(* Logix 5000 AddOnInstructionDefinition export EH_Micropilot_FMR43_IOL; software revision 38.00 *)

TYPE EH_CommAOI_Data :
STRUCT
   Device_Comm_Error : BOOL;
   CommSuccess : BOOL;
   CommFailed : BOOL;
   CommTimeOut : BOOL;
   StateDone : BOOL;
   NewState : BOOL;
   OldState : SINT;
   PortSize : SINT;
   DevicePort : SINT;
   MaxState : SINT;
   State : SINT;
   VendorID : INT;
   DeviceID : DINT;
   CyclicData : INT[16];
   AcyclicData : DINT[8];
   ReplayIndex : INT;
   AOI_Diagnostic : DINT;
   ConnectionStatus : DINT;
   OutputData : INT[16];
END_STRUCT
END_TYPE

ADD_ON_INSTRUCTION EH_Micropilot_FMR43_IOL   (* revision 1.2, vendor Endress+Hauser *)
// Micropilot FMR 43  Rev 1 IO-Link
// Revision note:
// 1.2 Added HeartbeatVerification, fixed Foamfunction
// 1.1 Changed the Datatype from Unsigned to Signed
// Add Disconnect check
VAR_IN_OUT
   DataToSend : INT[10]; {required}
   CommAOIBusy : DINT; {required}
   ActiveComPort : DINT; {required}
   DeviceAOISendRequest : DINT; {required}
   CommError : INT; {required}
   DeviceData : EH_CommAOI_Data; {required}
END_VAR
VAR_INPUT
   iSetSimulation : BOOL; {visible}
   iSimulationVariable : INT; {visible}
   iSimulationValue_Level : REAL; {visible}
   iSimulationValue_Distance : REAL; {visible}
   iSetUnit : BOOL; {visible}
   iUnit : SINT; {visible}
   iFoamDetection_Update : BOOL; {visible}
   iStart_HeartbeatVerification : BOOL; {visible}
END_VAR
VAR_OUTPUT
   qVendor_ID : DINT; {access Read Only, visible}
   qDevice_ID : DINT; {access Read Only, visible}
   qLevelLinearized : REAL; {access None, visible}
   qDistance : REAL; {visible}
   qExtendedDeviceStatus : INT; {access Read Only, visible}
   qUnit : SINT; {access Read Only, visible}
   qFoamIndex : REAL; {access Read Only, visible}
   qFoamDetected : BOOL; {access Read Only, visible}
   qBuildupIndex : REAL; {access Read Only, visible}
   qBuildupDetected : BOOL; {access Read Only, visible}
   qSSC1_1 : BOOL; {access Read Only, visible}
   qSSC1_2 : BOOL; {access Read Only, visible}
   qSSC2_1 : BOOL; {access Read Only, visible}
   qSSC2_2 : BOOL; {access Read Only, visible}
   qVerificationID : INT; {visible}
   qPassed : BOOL; {visible}
   qFailed : BOOL; {visible}
   qAOI_Diagnostic : DINT; {access Read Only, visible}
END_VAR
VAR_IN_OUT
   qAOI_Diagnostic_String : STRING; {required}
END_VAR
VAR_OUTPUT
   qActual_Diagnostics_Code : DINT; {access Read Only, visible}
END_VAR
VAR_IN_OUT
   qActual_Diagnostics_String : STRING; {required}
END_VAR
VAR_OUTPUT
   qLast_Diagnostics_Code : DINT; {visible}
END_VAR
VAR_IN_OUT
   qLast_Diagnostics_String : STRING; {required}
END_VAR
VAR_OUTPUT
   qCommError : DINT; {access None}
   qCommunicationBusy : DINT; {access Read Only, visible}
   qDeviceConnectionError : BOOL; {access Read Only, visible}
END_VAR
VAR
   Temp_DINT : DINT; {access None}
   CMD_Index : INT; {access None}
   CMD_Subindex : INT; {access None}
   CMD_ByteLength : INT; {access None}
   oldCondStatus : INT; {access None}
   oldSetSimulation : SINT; {access None}
   SetSimulation : SINT; {access None}
   SetUnit : SINT; {access None}
   oldSetUnit : SINT; {access None}
   Trigger : BOOL; {access None}
   CMD_Rd : BOOL; {access None}
   CMD_Wr : BOOL; {access None}
   SimulationDINT : DINT; {access None}
   InputByteLength : DINT; {access None}
   AOI_Prio : BOOL; {access None}
   StateMin : DINT; {access None}
   firstTimeDone : BOOL; {access None}
   OldStatus : DINT; {access None}
   CondStatusChanged : BOOL; {access None}
   Calc_ExtendedDeviceStatus : DINT; {access None}
   Totalizer1_DINT : DINT; {access None}
   SimActive : BOOL; {access None}
   CondStatusActive : BOOL; {access None}
   ActiveAOI : BOOL; {access None}
   Skip : BOOL; {access None}
   SimChanged : BOOL; {access None}
   UnitActive : BOOL; {access None}
   UnitChanged : BOOL; {access None}
   DeviceID : DINT; {access None}
   Calc_LevelLin : DINT; {access None}
   Calc_Distance : DINT; {access None}
   FALSE : BOOL; {access None}
   TRUE : BOOL := 1; {access None}
   temp_string1 : STRING; {access None}
   temp_string2 : STRING; {access None}
   qFoamIndexDINT : DINT; {access None}
   qFoamDetectedDINT : DINT; {access None}
   qBuildupIndexDINT : DINT; {access None}
   qBuildupDetectedDINT : DINT; {access None}
   qFoamDetectedREAL : REAL; {access None}
   qBuildupDetectedREAL : REAL; {access None}
   qLevelLinearizedTemp : REAL; {access None}
   TempLevel_DINT : DINT; {access None}
   TempDistance_DINT : DINT; {access None}
   qDistanceTemp : REAL; {access None}
   init : BOOL; {access None}
   SkipStep2 : BOOL; {access None}
   rTempLevel : REAL; {access None}
   rTempDistance : REAL;
   Start_HeartbeatVerification : SINT; {access None}
   oldStart_HeartbeatVerification : SINT; {access None}
   HeartbeatVerificationChanged : BOOL; {access None}
   HeartbeatVerificationActive : BOOL; {access None}
END_VAR

ROUTINE Logic   (* structured text *)
// Picomag Communication via AL1323
   // =======================================================================
   // Endress+Hauser Digital Solutions
   // ©Copyright (2024) All Rights Reserved
   // =======================================================================
   // Name:                EH_Micropilot_FMR43_IOL
   // Version:             1.2
   // Datum:               11.2025
   // Library:             01.01.00
   // Engineering:         Studio5000 V38.00.00
   // Author:              EH
   // =======================================================================
   
   qAOI_Diagnostic := DeviceData.AOI_Diagnostic;
   qCommunicationBusy := CommAOIBusy;
   DeviceID := 9553409;
   StateMin := 0;
   DeviceData.MaxState := 98;
   
   if DeviceData.DevicePort = 0 or DeviceData.DeviceID <> DeviceID or DeviceData.ConnectionStatus <> 1 then
   
   	qVendor_ID := DeviceData.VendorID;
   	qDevice_ID := DeviceData.DeviceID;
   	qLevelLinearized	:= 0;
   	qDistance	:= 0;
   	qExtendedDeviceStatus	:= 0;
   	qUnit	:= 0;
   	qFoamIndex := 0;   // Foam index
   	qFoamDetected := FALSE;   // Foam detection - TRUE if foam detected
   	qBuildupIndex := 0;   // Buildup index
   	qBuildupDetected := FALSE;   // Buildup detection - TRUE if buildup detected
   	qSSC1_1	:= FALSE;
   	qSSC1_2	:= FALSE;
   	qSSC2_1	:= FALSE;
   	qSSC2_2	:= FALSE;
   	qPassed := FALSE;
   	qFailed := FALSE;
   	qVerificationID := 0;
   	qPassed := FALSE;
   	qFailed	:= FALSE;
   	qActual_Diagnostics_Code	:= 0;
   	qLast_Diagnostics_Code	:= 0;
   	qLast_Diagnostics_String	:= '';
   	oldCondStatus := 0;
   	CondStatusChanged := FALSE;
   	init := FALSE;
   
   	if DeviceData.DevicePort = 0 then
   
   		qActual_Diagnostics_String	:= 'Device Port is Zero';
   		DeviceData.AOI_Diagnostic.1 := TRUE;
   
   	elsif DeviceData.ConnectionStatus <> 1 then
   
   		qActual_Diagnostics_String	:= 'No Device connected';
   		qDeviceConnectionError := TRUE;
   
   	elsif DeviceData.DeviceID <> DeviceID then
   
   		qActual_Diagnostics_String	:= 'Wrong DeviceID';
   		DeviceData.AOI_Diagnostic.2 := TRUE;
   	end_if;
   
   else
   
   	if qActual_Diagnostics_Code = 0  then
   
   		qActual_Diagnostics_String	:= '--------';
   
   	end_if;
   
   	if qLast_Diagnostics_Code = 0 then
   
   		qLast_Diagnostics_String	:= '--------';
   
   	end_if;
   
   	DeviceData.AOI_Diagnostic.1 := FALSE;
   	qDeviceConnectionError := FALSE;
   	DeviceData.AOI_Diagnostic.2  := FALSE;
   
   end_if;
   
   // Case device disconnected during communication to avoid blocking the communication
   if (DeviceData.AOI_Diagnostic.0 or qDeviceConnectionError or DeviceData.AOI_Diagnostic.2) and ActiveAOI and ActiveComPort = DeviceData.DevicePort and CommAOIBusy = 1 then
   
   	DeviceData.State := 0;
   	CommAOIBusy := 0;
   	DeviceAOISendRequest.[DeviceData.DevicePort] := 0;
   	ActiveComPort := 0;
   	ActiveAOI := 0;
   	DataToSend[0] := 0;
   	DataToSend[1] := 0;
   	DataToSend[2] := 0;
   	DataToSend[3] := 0;
   	DataToSend[4] := 0;
   	DataToSend[5] := 0;
   	DataToSend[6] := 0;
   	DataToSend[7] := 0;
   	DataToSend[8] := 0;
   	DataToSend[9] := 0;
   	DeviceData.StateDone := FALSE;
   	DeviceData.NewState := FALSE;
   	DeviceData.OldState := 0;
   	ActiveAOI := FALSE;
   
   end_if;
   
   if not DeviceData.AOI_Diagnostic.0
   	and not qDeviceConnectionError
   	and not DeviceData.AOI_Diagnostic.2
   	and DeviceData.DevicePort > 0 then
   
   	//*********************************
   	//Vendor ID
   	//*********************************
   
   		qVendor_ID := DeviceData.VendorID;
   
   	//*********************************
   	//Device ID
   	//*********************************
   
   		qDevice_ID := DeviceData.DeviceID;
   
   	//*********************************
   	// FMR43
   	//*********************************
   
   		Calc_LevelLin				:= 0;
   		Calc_Distance				:= 2;
   		Calc_ExtendedDeviceStatus	:= 4;
   
   	//*********************************
   	//Process Data Level Linearized
   	//*********************************
   
   		TempLevel_DINT	 := DeviceData.CyclicData[Calc_LevelLin+1];
   		TempLevel_DINT.8	 := DeviceData.CyclicData[Calc_LevelLin+1].8;
   		TempLevel_DINT.9  := DeviceData.CyclicData[Calc_LevelLin+1].9;
   		TempLevel_DINT.10 := DeviceData.CyclicData[Calc_LevelLin+1].10;
   		TempLevel_DINT.11 := DeviceData.CyclicData[Calc_LevelLin+1].11;
   		TempLevel_DINT.12 := DeviceData.CyclicData[Calc_LevelLin+1].12;
   		TempLevel_DINT.13 := DeviceData.CyclicData[Calc_LevelLin+1].13;
   		TempLevel_DINT.14 := DeviceData.CyclicData[Calc_LevelLin+1].14;
   		TempLevel_DINT.15 := DeviceData.CyclicData[Calc_LevelLin+1].15;
   		TempLevel_DINT.16 := DeviceData.CyclicData[Calc_LevelLin].0;
   		TempLevel_DINT.17 := DeviceData.CyclicData[Calc_LevelLin].1;
   		TempLevel_DINT.18 := DeviceData.CyclicData[Calc_LevelLin].2;
   		TempLevel_DINT.19 := DeviceData.CyclicData[Calc_LevelLin].3;
   		TempLevel_DINT.20 := DeviceData.CyclicData[Calc_LevelLin].4;
   		TempLevel_DINT.21 := DeviceData.CyclicData[Calc_LevelLin].5;
   		TempLevel_DINT.22 := DeviceData.CyclicData[Calc_LevelLin].6;
   		TempLevel_DINT.23 := DeviceData.CyclicData[Calc_LevelLin].7;
   		TempLevel_DINT.24 := DeviceData.CyclicData[Calc_LevelLin].8;
   		TempLevel_DINT.25 := DeviceData.CyclicData[Calc_LevelLin].9;
   		TempLevel_DINT.26 := DeviceData.CyclicData[Calc_LevelLin].10;
   		TempLevel_DINT.27 := DeviceData.CyclicData[Calc_LevelLin].11;
   		TempLevel_DINT.28 := DeviceData.CyclicData[Calc_LevelLin].12;
   		TempLevel_DINT.29 := DeviceData.CyclicData[Calc_LevelLin].13;
   		TempLevel_DINT.30 := DeviceData.CyclicData[Calc_LevelLin].14;
   		TempLevel_DINT.31 := DeviceData.CyclicData[Calc_LevelLin].15;
   
   		COP(TempLevel_DINT,qLevelLinearizedTemp,1);
   
   	//*********************************
   	//Process Data Distance
   	//*********************************
   
   		TempDistance_DINT	 := DeviceData.CyclicData[Calc_Distance+1];
   		TempDistance_DINT.8	 := DeviceData.CyclicData[Calc_Distance+1].8;
   		TempDistance_DINT.9	 := DeviceData.CyclicData[Calc_Distance+1].9;
   		TempDistance_DINT.10 := DeviceData.CyclicData[Calc_Distance+1].10;
   		TempDistance_DINT.11 := DeviceData.CyclicData[Calc_Distance+1].11;
   		TempDistance_DINT.12 := DeviceData.CyclicData[Calc_Distance+1].12;
   		TempDistance_DINT.13 := DeviceData.CyclicData[Calc_Distance+1].13;
   		TempDistance_DINT.14 := DeviceData.CyclicData[Calc_Distance+1].14;
   		TempDistance_DINT.15 := DeviceData.CyclicData[Calc_Distance+1].15;
   		TempDistance_DINT.16 := DeviceData.CyclicData[Calc_Distance].0;
   		TempDistance_DINT.17 := DeviceData.CyclicData[Calc_Distance].1;
   		TempDistance_DINT.18 := DeviceData.CyclicData[Calc_Distance].2;
   		TempDistance_DINT.19 := DeviceData.CyclicData[Calc_Distance].3;
   		TempDistance_DINT.20 := DeviceData.CyclicData[Calc_Distance].4;
   		TempDistance_DINT.21 := DeviceData.CyclicData[Calc_Distance].5;
   		TempDistance_DINT.22 := DeviceData.CyclicData[Calc_Distance].6;
   		TempDistance_DINT.23 := DeviceData.CyclicData[Calc_Distance].7;
   		TempDistance_DINT.24 := DeviceData.CyclicData[Calc_Distance].8;
   		TempDistance_DINT.25 := DeviceData.CyclicData[Calc_Distance].9;
   		TempDistance_DINT.26 := DeviceData.CyclicData[Calc_Distance].10;
   		TempDistance_DINT.27 := DeviceData.CyclicData[Calc_Distance].11;
   		TempDistance_DINT.28 := DeviceData.CyclicData[Calc_Distance].12;
   		TempDistance_DINT.29 := DeviceData.CyclicData[Calc_Distance].13;
   		TempDistance_DINT.30 := DeviceData.CyclicData[Calc_Distance].14;
   		TempDistance_DINT.31 := DeviceData.CyclicData[Calc_Distance].15;
   
   		COP(TempDistance_DINT,qDistanceTemp,1);
   
   		case qUnit of
   
   				//*********************************
   				45: // m
   				//*********************************
   					qDistance := qDistanceTemp;
   					qLevelLinearized := qLevelLinearizedTemp;
   
   				//*********************************
   				47: // inch
   				//*********************************
   					qDistance := qDistanceTemp * 39.37007874;
   					qLevelLinearized := qLevelLinearizedTemp * 39.37007874;
   
   				//*********************************
   				49: // mm
   				//*********************************
   					qDistance := qDistanceTemp * 1000;
   					qLevelLinearized := qLevelLinearizedTemp * 1000;
   
   				else // Base unit
   					qDistance := qDistanceTemp;
   					qLevelLinearized := qLevelLinearizedTemp;
   
   			end_case;
   
   	//*********************************
   	// Extended device Status
   	//*********************************
   
   		qExtendedDeviceStatus.0 := DeviceData.CyclicData[Calc_ExtendedDeviceStatus].8;
   		qExtendedDeviceStatus.1 := DeviceData.CyclicData[Calc_ExtendedDeviceStatus].9;
   		qExtendedDeviceStatus.2 := DeviceData.CyclicData[Calc_ExtendedDeviceStatus].10;
   		qExtendedDeviceStatus.3 := DeviceData.CyclicData[Calc_ExtendedDeviceStatus].11;
   		qExtendedDeviceStatus.4 := DeviceData.CyclicData[Calc_ExtendedDeviceStatus].12;
   		qExtendedDeviceStatus.5 := DeviceData.CyclicData[Calc_ExtendedDeviceStatus].13;
   		qExtendedDeviceStatus.6 := DeviceData.CyclicData[Calc_ExtendedDeviceStatus].14;
   		qExtendedDeviceStatus.7 := DeviceData.CyclicData[Calc_ExtendedDeviceStatus].15;
   
   	//*********************************
   	// Process Parameter SSC
   	//*********************************
   
   		qSSC1_1 := DeviceData.CyclicData[Calc_ExtendedDeviceStatus].0;
   		qSSC1_2 := DeviceData.CyclicData[Calc_ExtendedDeviceStatus].1;
   
   		qSSC2_1 := DeviceData.CyclicData[Calc_ExtendedDeviceStatus].2;
   		qSSC2_2 := DeviceData.CyclicData[Calc_ExtendedDeviceStatus].3;
   
   	//*********************************
   	// Checking for Changed Status
   	//*********************************
   
   		SetSimulation.0 := iSetSimulation;
   		SetUnit.0 := iSetUnit;
   		Start_HeartbeatVerification.0 := iStart_HeartbeatVerification;
   
   	if oldCondStatus <> qExtendedDeviceStatus and not CondStatusChanged or iFoamDetection_Update and (qExtendedDeviceStatus = 120 or qExtendedDeviceStatus = 121) then
   
   		CondStatusChanged := TRUE;
   		oldCondStatus := qExtendedDeviceStatus;
   
   	end_if;
   
   	if oldSetSimulation <> SetSimulation and not SimChanged then
   
   		if oldSetSimulation < SetSimulation then
   
   			SimChanged := TRUE;
   
   		end_if;
   
   		oldSetSimulation := SetSimulation;
   
   	end_if;
   
   	if oldSetUnit <> SetUnit and not UnitChanged then
   
   		if oldSetUnit < SetUnit then
   
   			UnitChanged := TRUE;
   
   		end_if;
   
   		oldSetUnit := SetUnit;
   
   	end_if;
   
   	if oldStart_HeartbeatVerification <> Start_HeartbeatVerification and not HeartbeatVerificationChanged then
   
   		if oldStart_HeartbeatVerification < Start_HeartbeatVerification then
   
   			HeartbeatVerificationChanged := TRUE;
   
   		end_if;
   
   		oldStart_HeartbeatVerification := Start_HeartbeatVerification;
   
   	end_if;
   
   	if CondStatusChanged
   	and not ActiveAOI
   	and not CondStatusActive
   	and not Skip then
   
   		DeviceAOISendRequest.[DeviceData.DevicePort] := TRUE;
   		CondStatusActive := TRUE;
   		Skip := TRUE;
   
   	elsif SimChanged
   		and not ActiveAOI
   		and not SimActive
   		and not Skip then
   
   		DeviceAOISendRequest.[DeviceData.DevicePort] := TRUE;
   		SimActive := TRUE;
   		Skip := TRUE;
   
   	elsif HeartbeatVerificationChanged
   		and not ActiveAOI
   		and not HeartbeatVerificationActive
   		and not Skip then
   
   		DeviceAOISendRequest.[DeviceData.DevicePort] := TRUE;
   		HeartbeatVerificationActive := TRUE;
   		Skip := TRUE;
   
   	elsif UnitChanged
   		and not ActiveAOI
   		and not UnitActive
   		and not Skip then
   
   		DeviceAOISendRequest.[DeviceData.DevicePort] := TRUE;
   		UnitActive := TRUE;
   		Skip := TRUE;
   
   	end_if;
   
   	if ActiveComPort = DeviceData.DevicePort then
   
   		AOI_Prio := TRUE;
   
   	else
   
   		AOI_Prio := FALSE;
   
   	end_if;
   
   	if (SimActive or UnitActive or HeartbeatVerificationActive or CondStatusActive) and CommAOIBusy = 1  and DeviceData.State = 0 and AOI_Prio and not ActiveAOI then
   
   		ActiveAOI := TRUE;
   		Skip := FALSE;
   
   	end_if;
   
   	qCommunicationBusy := CommAOIBusy;
   	qAOI_Diagnostic :=DeviceData.AOI_Diagnostic;
   
   	//*********************************
   	// States for Execution
   	//*********************************
   
   	if ActiveAOI or DeviceData.State = DeviceData.MaxState then
   
   	case DeviceData.State of
   
   		//*********************************
   		0: // Idle
   		//*********************************
   
   			// Initializing
   			Trigger := 0;
   			CMD_Index := 0;
   			CMD_Subindex := 0;
   			CMD_Wr := FALSE;
   			CMD_Rd := FALSE;
   		    CMD_ByteLength := 0;
   
   			if DeviceData.DevicePort = ActiveComPort then
   					DeviceData.CommSuccess := FALSE;
   					DeviceData.CommTimeOut := FALSE;
   					DeviceData.NewState := TRUE;
   					DeviceData.StateDone := FALSE;
   				end_if;
   
   			// Wait for trigger
   			if SimActive then
   
   				DeviceData.AOI_Diagnostic := 0;
   				DeviceData.State := 1;
   
   			elsif UnitActive then
   
   				DeviceData.AOI_Diagnostic := 0;
   				DeviceData.State := 4;
   
   			elsif HeartbeatVerificationActive then
   
   				DeviceData.AOI_Diagnostic := 0;
   				DeviceData.State := 80;
   
   			elsif CondStatusChanged then
   
   				if not init then
   
   					DeviceData.State := 5;
   
   				else
   
   					DeviceData.State := 90;
   
   				end_if;
   
   			end_if;
   
   	//*********************************
   	1: // Set Simulation Variable
   	//*********************************
   
   			CMD_Index := 1332;
   			CMD_Subindex := 0;
   			CMD_Wr := TRUE;								// Only Read or Write can be active = 1
   			CMD_Rd := FALSE;
   			CMD_ByteLength := 2;
   			DataToSend[6]:= 0;
   			DataToSend[7]:= 0;
   
   			if iSimulationVariable > 0 then
   
   				DataToSend[6].8 := iSimulationVariable.0;
   				DataToSend[6].9 := iSimulationVariable.1;
   				DataToSend[6].10 := iSimulationVariable.2;
   				DataToSend[6].11 := iSimulationVariable.3;
   				DataToSend[6].12 := iSimulationVariable.4;
   				DataToSend[6].13 := iSimulationVariable.5;
   				DataToSend[6].14 := iSimulationVariable.6;
   				DataToSend[6].15 := iSimulationVariable.7;
   
   			else
   				DataToSend[6] := 0;
   				DataToSend[7] := 0;
   			end_if;
   
   			Trigger := TRUE;
   
   			if DeviceData.NewState then
   				DeviceData.StateDone := TRUE;
   			end_if;
   
   			if  DeviceData.CommSuccess and DeviceData.ReplayIndex = CMD_Index then
   
   				Trigger := FALSE;
   				DeviceData.OldState := DeviceData.State;
   				DeviceData.State := DeviceData.State + 1;
   				DeviceData.CommSuccess := FALSE;
   				DeviceData.AcyclicData[0] := 0;
   				DeviceData.NewState := TRUE;
   
   				elsif DeviceData.CommTimeOut then
   
   					temp_string1 := 'Error in step ';
   					Temp_DINT := DeviceData.State;
   					DTOS(Temp_DINT, temp_string2);
   					CONCAT(temp_string1, temp_string2, qAOI_Diagnostic_String);
   
   					DeviceData.OldState := DeviceData.State;
   					DeviceData.State := DeviceData.MaxState;
   					DeviceData.CommTimeOut := FALSE;
   					DeviceData.AcyclicData[0] := 0;
   					DeviceData.NewState := TRUE;
   
   			end_if;
   
   
   		//*********************************
   		2: // Set Simulation Value
   		//*********************************
   
   			CMD_Subindex := 0;
   			CMD_Wr := TRUE;								// Only Read or Write can be active = 1
   			CMD_Rd := FALSE;
   			CMD_ByteLength := 4;
   			DataToSend[6]:= 0;
   			DataToSend[7]:= 0;
   
   			case qUnit of
   
   				//*********************************
   				45: // m
   				//*********************************
   					rTempLevel := iSimulationValue_Level;
   					rTempDistance := iSimulationValue_Distance;
   
   				//*********************************
   				47: // inch
   				//*********************************
   
   					rTempLevel := iSimulationValue_Level / 39.37007874;
   					rTempDistance := iSimulationValue_Distance / 39.37007874;
   
   				//*********************************
   				49: // mm
   				//*********************************
   					rTempLevel := iSimulationValue_Level / 1000;
   					rTempDistance := iSimulationValue_Distance / 1000;
   
   			else // Base unit
   
   					rTempLevel := iSimulationValue_Level;
   					rTempDistance := iSimulationValue_Distance;
   
   			end_case;
   
   			CASE iSimulationVariable OF
   
   				1:
   					COP(rTempLevel,SimulationDINT,1); // Copy the Bits from the Real in a DINT
   					CMD_Index := 8213;
   				3:
   					COP(rTempDistance,SimulationDINT,1); // Copy the Bits from the Real in a DINT
   					CMD_Index := 8829;
   
   				else
   
   					SkipStep2 := TRUE;
   
   			END_CASE;
   
   			if not SkipStep2 then
   
   				DataToSend[6].0 :=  SimulationDINT.24;
   				DataToSend[6].1 :=  SimulationDINT.25;
   				DataToSend[6].2 :=  SimulationDINT.26;
   				DataToSend[6].3 :=  SimulationDINT.27;
   				DataToSend[6].4 :=  SimulationDINT.28;
   				DataToSend[6].5 :=  SimulationDINT.29;
   				DataToSend[6].6 :=  SimulationDINT.30;
   				DataToSend[6].7 :=  SimulationDINT.31;
   				DataToSend[6].8 :=  SimulationDINT.16;
   				DataToSend[6].9 :=  SimulationDINT.17;
   				DataToSend[6].10 := SimulationDINT.18;
   				DataToSend[6].11 := SimulationDINT.19;
   				DataToSend[6].12 := SimulationDINT.20;
   				DataToSend[6].13 := SimulationDINT.21;
   				DataToSend[6].14 := SimulationDINT.22;
   				DataToSend[6].15 := SimulationDINT.23;
   				DataToSend[7].0  := SimulationDINT.8;
   				DataToSend[7].1  := SimulationDINT.9;
   				DataToSend[7].2  := SimulationDINT.10;
   				DataToSend[7].3  := SimulationDINT.11;
   				DataToSend[7].4  := SimulationDINT.12;
   				DataToSend[7].5  := SimulationDINT.13;
   				DataToSend[7].6  := SimulationDINT.14;
   				DataToSend[7].7  := SimulationDINT.15;
   				DataToSend[7].8  := SimulationDINT.0;
   				DataToSend[7].9  := SimulationDINT.1;
   				DataToSend[7].10 := SimulationDINT.2;
   				DataToSend[7].11 := SimulationDINT.3;
   				DataToSend[7].12 := SimulationDINT.4;
   				DataToSend[7].13 := SimulationDINT.5;
   				DataToSend[7].14 := SimulationDINT.6;
   				DataToSend[7].15 := SimulationDINT.7;
   
   				Trigger := TRUE;
   
   				if DeviceData.NewState then
   					DeviceData.StateDone := TRUE;
   				end_if;
   
   				if  DeviceData.CommSuccess and DeviceData.ReplayIndex = CMD_Index then
   
   					Trigger := FALSE;
   					DeviceData.OldState := DeviceData.State;
   					DeviceData.State := DeviceData.MaxState;
   					DeviceData.CommSuccess := FALSE;
   					DeviceData.AcyclicData[0] := 0;
   					DeviceData.NewState := TRUE;
   
   				elsif DeviceData.CommTimeOut then
   
   					temp_string1 := 'Error in step ';
   					Temp_DINT := DeviceData.State;
   					DTOS(Temp_DINT, temp_string2);
   					CONCAT(temp_string1, temp_string2, qAOI_Diagnostic_String);
   
   					DeviceData.OldState := DeviceData.State;
   					DeviceData.State := DeviceData.MaxState;
   					DeviceData.CommTimeOut := FALSE;
   					DeviceData.AcyclicData[0] := 0;
   					DeviceData.NewState := TRUE;
   
   				end_if;
   
   			else
   
   
   					temp_string1 := 'Error in step ';
   					Temp_DINT := DeviceData.State;
   					DTOS(Temp_DINT, temp_string2);
   					CONCAT(temp_string1, temp_string2, qAOI_Diagnostic_String);
   
   					DeviceData.OldState := DeviceData.State;
   					DeviceData.State := DeviceData.MaxState;
   					DeviceData.CommTimeOut := FALSE;
   					DeviceData.AcyclicData[0] := 0;
   					DeviceData.NewState := TRUE;
   					SkipStep2 := FALSE;
   			end_if;
   
   		//*********************************
   		4: // Set unit
   		//*********************************
   
   			CMD_Index := 321;
   			CMD_Subindex := 0;
   			CMD_Wr := TRUE;								// Only Read or Write can be active = 1
   			CMD_Rd := FALSE;
   			CMD_ByteLength := 2;
   			DataToSend[6] := 0;
   			DataToSend[7] := 0;
   
   			if iUnit = 45 OR iUnit = 47 OR iUnit = 49 then
   
   				DataToSend[6].8 := iUnit.0;
   				DataToSend[6].9 := iUnit.1;
   				DataToSend[6].10 := iUnit.2;
   				DataToSend[6].11 := iUnit.3;
   				DataToSend[6].12 := iUnit.4;
   				DataToSend[6].13 := iUnit.5;
   				DataToSend[6].14 := iUnit.6;
   				DataToSend[6].15 := iUnit.7;
   
   				Trigger := TRUE;
   
   				if DeviceData.NewState then
   					DeviceData.StateDone := TRUE;
   				end_if;
   
   				if  DeviceData.CommSuccess and DeviceData.ReplayIndex = CMD_Index then
   
   					Trigger := FALSE;
   					DeviceData.OldState := DeviceData.State;
   					DeviceData.State := DeviceData.State + 1;
   					DeviceData.CommSuccess := FALSE;
   					DeviceData.AcyclicData[0] := 0;
   					DeviceData.NewState := TRUE;
   
   			 	elsif DeviceData.CommTimeOut then
   
   					temp_string1 := 'Error in step ';
   					Temp_DINT := DeviceData.State;
   					DTOS(Temp_DINT, temp_string2);
   					CONCAT(temp_string1, temp_string2, qAOI_Diagnostic_String);
   
   					DeviceData.OldState := DeviceData.State;
   					DeviceData.State := DeviceData.MaxState;	//Check State
   					DeviceData.CommTimeOut := FALSE;
   					DeviceData.AcyclicData[0] := 0;
   					DeviceData.NewState := TRUE;
   
   				end_if;
   
   			else
   
   					temp_string1 := 'Error in step ';
   					Temp_DINT := DeviceData.State;
   					DTOS(Temp_DINT, temp_string2);
   					CONCAT(temp_string1, temp_string2, qAOI_Diagnostic_String);
   
   					DeviceData.OldState := DeviceData.State;
   					DeviceData.State := DeviceData.MaxState;
   					DeviceData.CommTimeOut := FALSE;
   					DeviceData.AcyclicData[0] := 0;
   					DeviceData.NewState := TRUE;
   
   	        end_if;
   
   		//*********************************
   		5: // Read Unit
   		//*********************************
   
   				CMD_Index := 321;
   				CMD_Subindex := 0;
   				CMD_Wr := FALSE;
   				CMD_Rd := TRUE;
   				CMD_ByteLength := 2;
   				Trigger := TRUE;
   
   				if DeviceData.NewState then
   					DeviceData.StateDone := TRUE;
   				end_if;
   
   				if  DeviceData.CommSuccess and DeviceData.ReplayIndex = CMD_Index then
   
   					qUnit.0	:= DeviceData.AcyclicData[0].0;
   					qUnit.1	:= DeviceData.AcyclicData[0].1;
   					qUnit.2	:= DeviceData.AcyclicData[0].2;
   					qUnit.3	:= DeviceData.AcyclicData[0].3;
   					qUnit.4	:= DeviceData.AcyclicData[0].4;
   					qUnit.5	:= DeviceData.AcyclicData[0].5;
   					qUnit.6	:= DeviceData.AcyclicData[0].6;
   					qUnit.7	:= DeviceData.AcyclicData[0].7;
   
   					Trigger := FALSE;
   					DeviceData.OldState := DeviceData.State;
   					DeviceData.State := DeviceData.MaxState;
   					DeviceData.CommSuccess := FALSE;
   					DeviceData.AcyclicData[0] := 0;
   					DeviceData.NewState := TRUE;
   
   					if not init then
   
   						init := TRUE;
   						DeviceData.State := 90;
   
   					end_if;
   
   				 elsif DeviceData.CommTimeOut then
   
   					temp_string1 := 'Error in step ';
   					Temp_DINT := DeviceData.State;
   					DTOS(Temp_DINT, temp_string2);
   					CONCAT(temp_string1, temp_string2, qAOI_Diagnostic_String);
   
   					DeviceData.OldState := DeviceData.State;
   					DeviceData.State := DeviceData.MaxState;
   					DeviceData.CommTimeOut := FALSE;
   					DeviceData.AcyclicData[0] := 0;
   					DeviceData.NewState := TRUE;
   
   				end_if;
   
   		//*********************************
   		80: // Check Heartbeat Verification activation
   		//*********************************
   			CMD_Index := 12342;
   			CMD_Subindex := 0;
   			CMD_Wr := FALSE;
   			CMD_Rd := TRUE;
   			CMD_ByteLength := 1;
   			Trigger := TRUE;
   			DataToSend[6]:= 0;
   			DataToSend[7]:= 0;
   
   			if DeviceData.NewState then
   
   				DeviceData.StateDone := TRUE;
   
   			end_if;
   
   			if  DeviceData.CommSuccess and DeviceData.ReplayIndex = CMD_Index then
   
   				if DeviceData.AcyclicData[0] = 1 then
   
   					DeviceData.State := DeviceData.State + 1;
   
   				else
   					qAOI_Diagnostic_String := 'Step 80: Software Option not activated ';
   
   					DeviceData.OldState := DeviceData.State;
   					DeviceData.State := DeviceData.MaxState;
   
   				end_if;
   
   				Trigger := FALSE;
   				DeviceData.CommSuccess := FALSE;
   				DeviceData.AcyclicData[0] := 0;
   				DeviceData.NewState := TRUE;
   
   			 elsif DeviceData.CommTimeOut then
   
   				temp_string1 := 'Error in step ';
   				Temp_DINT := DeviceData.State;
   				DTOS(Temp_DINT, temp_string2);
   				CONCAT(temp_string1, temp_string2, qAOI_Diagnostic_String);
   
   				DeviceData.OldState := DeviceData.State;
   				DeviceData.State := DeviceData.MaxState;
   				DeviceData.CommTimeOut := FALSE;
   				DeviceData.AcyclicData[0] := 0;
   				DeviceData.NewState := TRUE;
   
   			end_if;
   
   		//*********************************
   		81: // Check if Verifivation is ongoing
   		//*********************************
   			CMD_Index := 12323;
   			CMD_Subindex := 0;
   			CMD_Wr := FALSE;
   			CMD_Rd := TRUE;
   			CMD_ByteLength := 2;
   			Trigger := TRUE;
   
   			if DeviceData.NewState then
   
   				DeviceData.StateDone := TRUE;
   
   			end_if;
   
   			if  DeviceData.CommSuccess and DeviceData.ReplayIndex = CMD_Index then
   
   				if DeviceData.AcyclicData[0] <> 8 then
   
   					DeviceData.State := DeviceData.State + 1;
   
   				else
   					qAOI_Diagnostic_String := 'Step 81: Heartbeat Verification already in progress ';
   					DeviceData.OldState := DeviceData.State;
   					DeviceData.State := DeviceData.MaxState;
   					DeviceData.CommTimeOut := FALSE;
   
   				end_if;
   
   				Trigger := FALSE;
   				DeviceData.CommSuccess := FALSE;
   				DeviceData.AcyclicData[0] := 0;
   				DeviceData.NewState := TRUE;
   
   			 elsif DeviceData.CommTimeOut then
   
   				temp_string1 := 'Error in step ';
   				Temp_DINT := DeviceData.State;
   				DTOS(Temp_DINT, temp_string2);
   				CONCAT(temp_string1, temp_string2, qAOI_Diagnostic_String);
   
   				DeviceData.OldState := DeviceData.State;
   				DeviceData.State := DeviceData.MaxState;
   				DeviceData.CommTimeOut := FALSE;
   				DeviceData.AcyclicData[0] := 0;
   				DeviceData.NewState := TRUE;
   
   			end_if;
   
   		//*********************************
   		82: // Start Verification
   		//*********************************
   			CMD_Index := 12325;
   			CMD_Subindex := 0;
   			CMD_Wr := TRUE;
   			CMD_Rd := FALSE;
   			CMD_ByteLength := 2;
   			Trigger := TRUE;
   			DataToSend[6] := 0;
   			DataToSend[7] := 0;
   
   			DataToSend[6].8 := TRUE;
   
   			if DeviceData.NewState then
   
   				DeviceData.StateDone := TRUE;
   
   			end_if;
   
   		if DeviceData.CommSuccess and DeviceData.ReplayIndex = CMD_Index then
   
   		    Trigger := FALSE;
   		    DeviceData.CommSuccess := FALSE;
   		    DeviceData.State := DeviceData.State + 3;
   			DeviceData.AcyclicData[0] := 0;
   			DeviceData.NewState := TRUE;
   
   		elsif DeviceData.CommTimeOut then
   
   		    temp_string1 := 'Error in step ';
   		    Temp_DINT := DeviceData.State;
   		    DTOS(Temp_DINT, temp_string2);
   		    CONCAT(temp_string1, temp_string2, qAOI_Diagnostic_String);
   
   		    DeviceData.OldState := DeviceData.State;
   		    DeviceData.State := DeviceData.MaxState;
   		    DeviceData.CommTimeOut := FALSE;
   			DeviceData.AcyclicData[0] := 0;
   			DeviceData.NewState := TRUE;
   
   		end_if;
   
   
   		//*********************************
   		83: // Intermediate state
   		//*********************************
   			CMD_Index := 36;
   			CMD_Subindex := 0;
   			CMD_Wr := FALSE;
   			CMD_Rd := TRUE;
   			CMD_ByteLength := 1;
   			Trigger := TRUE;
   
   			if DeviceData.NewState then
   
   				DeviceData.StateDone := TRUE;
   
   			end_if;
   
   			if DeviceData.CommSuccess and DeviceData.ReplayIndex = CMD_Index then
   
   			    DeviceData.State := DeviceData.State + 2;
   			    Trigger := FALSE;
   			    DeviceData.CommSuccess := FALSE;
   				DeviceData.AcyclicData[0] := 0;
   				DeviceData.NewState := TRUE;
   
   			elsif DeviceData.CommTimeOut then
   
   			    temp_string1 := 'Error in step ';
   			    Temp_DINT := DeviceData.State;
   			    DTOS(Temp_DINT, temp_string2);
   			    CONCAT(temp_string1, temp_string2, qAOI_Diagnostic_String);
   
   			    DeviceData.OldState := DeviceData.State;
   			    DeviceData.State := DeviceData.MaxState;
   			    DeviceData.CommTimeOut := FALSE;
   				DeviceData.AcyclicData[0] := 0;
   				DeviceData.NewState := TRUE;
   
   			end_if;
   
   		//*********************************
   		84: // Read progress
   		//*********************************
   
   		//*********************************
   		85: // Read status
   		//*********************************
   			CMD_Index := 12323;
   			CMD_Subindex := 0;
   			CMD_Wr := FALSE;
   			CMD_Rd := TRUE;
   			CMD_ByteLength := 2;
   			Trigger := TRUE;
   
   			if DeviceData.NewState then
   
   				DeviceData.StateDone := TRUE;
   
   			end_if;
   
   			if DeviceData.CommSuccess and DeviceData.ReplayIndex = CMD_Index then
   
   			    if DeviceData.AcyclicData[0] = 10 then
   
   			        DeviceData.State := DeviceData.State + 1;
   
   			    elsif DeviceData.AcyclicData[0] = 8 then
   
   					DeviceData.State := DeviceData.State - 2;
   
   			    else
   			        qAOI_Diagnostic_String := 'Step 85: Heartbeat Verification not done';
   			        DeviceData.OldState := DeviceData.State;
   			        DeviceData.State := DeviceData.MaxState;
   			        DeviceData.CommTimeOut := FALSE;
   
   			    end_if;
   
   			    Trigger := FALSE;
   			    DeviceData.CommSuccess := FALSE;
   				DeviceData.AcyclicData[0] := 0;
   				DeviceData.NewState := TRUE;
   
   			elsif DeviceData.CommTimeOut then
   
   			    temp_string1 := 'Error in step ';
   			    Temp_DINT := DeviceData.State;
   			    DTOS(Temp_DINT, temp_string2);
   			    CONCAT(temp_string1, temp_string2, qAOI_Diagnostic_String);
   
   			    DeviceData.OldState := DeviceData.State;
   			    DeviceData.State := DeviceData.MaxState;
   			    DeviceData.CommTimeOut := FALSE;
   				DeviceData.AcyclicData[0] := 0;
   				DeviceData.NewState := TRUE;
   
   			end_if;
   
   		//*********************************
   		86: // Read overall result
   		//*********************************
   			CMD_Index := 1396;
   			CMD_Subindex := 0;
   			CMD_Wr := FALSE;
   			CMD_Rd := TRUE;
   			CMD_ByteLength := 2;
   			Trigger := TRUE;
   
   			if DeviceData.NewState then
   
   				DeviceData.StateDone := TRUE;
   
   			end_if;
   
   			if  DeviceData.CommSuccess and DeviceData.ReplayIndex = CMD_Index then
   
   				if DeviceData.AcyclicData[0] = 1 then
   
   					qPassed := TRUE;
   					qFailed := FALSE;
   
   				else
   
   					qPassed := FALSE;
   					qFailed := TRUE;
   
   				end_if;
   
   				Trigger := FALSE;
   				DeviceData.CommSuccess := FALSE;
   				DeviceData.State := DeviceData.State + 1;
   				DeviceData.AcyclicData[0] := 0;
   				DeviceData.NewState := TRUE;
   
   			 elsif DeviceData.CommTimeOut then
   
   				temp_string1 := 'Error in step ';
   				Temp_DINT := DeviceData.State;
   				DTOS(Temp_DINT, temp_string2);
   				CONCAT(temp_string1, temp_string2, qAOI_Diagnostic_String);
   
   				DeviceData.CommTimeOut := FALSE;
   				DeviceData.OldState := DeviceData.State;
   				DeviceData.State := DeviceData.MaxState;
   				DeviceData.AcyclicData[0] := 0;
   				DeviceData.NewState := TRUE;
   
   			end_if;
   
   		//*********************************
   		87: // Read Verification ID
   		//*********************************
   			CMD_Index := 12321;
   			CMD_Subindex := 0;
   			CMD_Wr := FALSE;
   			CMD_Rd := TRUE;
   			CMD_ByteLength := 2;
   			Trigger := TRUE;
   
   			if DeviceData.NewState then
   
   				DeviceData.StateDone := TRUE;
   
   			end_if;
   
   			if  DeviceData.CommSuccess and DeviceData.ReplayIndex = CMD_Index then
   
   				qVerificationID.0	:= DeviceData.AcyclicData[0].0;
   				qVerificationID.1	:= DeviceData.AcyclicData[0].1;
   				qVerificationID.2	:= DeviceData.AcyclicData[0].2;
   				qVerificationID.3	:= DeviceData.AcyclicData[0].3;
   				qVerificationID.4	:= DeviceData.AcyclicData[0].4;
   				qVerificationID.5	:= DeviceData.AcyclicData[0].5;
   				qVerificationID.6	:= DeviceData.AcyclicData[0].6;
   				qVerificationID.7	:= DeviceData.AcyclicData[0].7;
   				qVerificationID.8	:= DeviceData.AcyclicData[0].8;
   				qVerificationID.9	:= DeviceData.AcyclicData[0].9;
   				qVerificationID.10	:= DeviceData.AcyclicData[0].10;
   				qVerificationID.11	:= DeviceData.AcyclicData[0].11;
   				qVerificationID.12	:= DeviceData.AcyclicData[0].12;
   				qVerificationID.13	:= DeviceData.AcyclicData[0].13;
   				qVerificationID.14	:= DeviceData.AcyclicData[0].14;
   				qVerificationID.15	:= DeviceData.AcyclicData[0].15;
   
   				Trigger := FALSE;
   				DeviceData.CommSuccess := FALSE;
   				DeviceData.OldState := DeviceData.State;
   				DeviceData.State := DeviceData.MaxState;
   				DeviceData.NewState := TRUE;
   
   			 elsif DeviceData.CommTimeOut then
   
   				temp_string1 := 'Error in step ';
   				Temp_DINT := DeviceData.State;
   				DTOS(Temp_DINT, temp_string2);
   				CONCAT(temp_string1, temp_string2, qAOI_Diagnostic_String);
   
   				DeviceData.CommTimeOut := FALSE;
   				DeviceData.OldState := DeviceData.State;
   				DeviceData.State := DeviceData.MaxState;
   				DeviceData.NewState := TRUE;
   
   			end_if;
   
   		//*********************************
   		90: // Actual Diagnostic
   		//*********************************
   
   			CMD_Index := 297;
   			CMD_Subindex := 0;
   			CMD_Wr := FALSE;
   			CMD_Rd := TRUE;
   			CMD_ByteLength := 4;
   			Trigger := TRUE;
   
   			if DeviceData.NewState then
   				DeviceData.StateDone := 1;
   			end_if;
   
   			if  DeviceData.CommSuccess and DeviceData.ReplayIndex = CMD_Index then
   
   				qActual_Diagnostics_Code	:= DeviceData.AcyclicData[0];
   
   				case qActual_Diagnostics_Code of
   
   					0:
   						qActual_Diagnostics_String := '--------';
   					16777250:
   						qActual_Diagnostics_String := 'F062 Sensor connection faulty';
   					16777259:
   						qActual_Diagnostics_String := 'F801 Supply voltage too low';
   					16777267:
   						qActual_Diagnostics_String := 'F435 Linearization faulty';
   					16777283:
   						qActual_Diagnostics_String := 'F803 Loop current faulty';
   					16777310:
   						qActual_Diagnostics_String := 'F942 In safety distance';
   					16777312:
   						qActual_Diagnostics_String := 'F437 Configuration incompatible';
   					16777314:
   						qActual_Diagnostics_String := 'F282 Data storage inconsistent';
   					16777319:
   						qActual_Diagnostics_String := 'F242 Firmware incompatible';
   					16777323:
   						qActual_Diagnostics_String := 'F252 Module incompatible';
   					16777325:
   						qActual_Diagnostics_String := 'F270 Main electronics defective';
   					16777334:
   						qActual_Diagnostics_String := 'F941 Echo lost';
   					16777336:
   						qActual_Diagnostics_String := 'F270 Main electronics defective';
   					16777337:
   						qActual_Diagnostics_String := 'F272 Main electronics faulty';
   					16777340:
   						qActual_Diagnostics_String := 'F270 Main electronics defective';
   					16777341:
   						qActual_Diagnostics_String := 'F272 Main electronics faulty';
   					16777343:
   						qActual_Diagnostics_String := 'F270 Main electronics defective';
   					16777344:
   						qActual_Diagnostics_String := 'F270 Main electronics defective';
   					16777348:
   						qActual_Diagnostics_String := 'F270 Main electronics defective';
   					16777355:
   						qActual_Diagnostics_String := 'F410 Data transfer failed';
   					16777374:
   						qActual_Diagnostics_String := 'F283 Memory content inconsistent';
   					16777375:
   						qActual_Diagnostics_String := 'F270 Main electronics defective';
   					16777387:
   						qActual_Diagnostics_String := 'F270 Main electronics defective';
   					16777388:
   						qActual_Diagnostics_String := 'F151 Sensor electronic failure';
   					16777389:
   						qActual_Diagnostics_String := 'F805 Loop current faulty';
   					16777390:
   						qActual_Diagnostics_String := 'F151 Sensor electronic failure';
   					16777396:
   						qActual_Diagnostics_String := 'F151 Sensor electronic failure';
   					16777399:
   						qActual_Diagnostics_String := 'F151 Sensor electronic failure';
   					16777441:
   						qActual_Diagnostics_String := 'F283 Memory content inconsistent';
   					16777445:
   						qActual_Diagnostics_String := 'F273 Main electronics defective';
   					16777446:
   						qActual_Diagnostics_String := 'F388 Electronics and HistoROM defective';
   					16777816:
   						qActual_Diagnostics_String := 'F272 Main electronics faulty';
   					16777817:
   						qActual_Diagnostics_String := 'F151 Sensor electronic failure';
   					16777818:
   						qActual_Diagnostics_String := 'F151 Sensor electronic failure';
   					16777885:
   						qActual_Diagnostics_String := 'F151 Sensor electronic failure';
   					16777886:
   						qActual_Diagnostics_String := 'F151 Sensor electronic failure';
   					16778096:
   						qActual_Diagnostics_String := 'F168 Buildup detected';
   					16778097:
   						qActual_Diagnostics_String := 'F952 Foam detected';
   					16778191:
   						qActual_Diagnostics_String := 'F538 Configuration Sensor Unit invalid';
   					16778253:
   						qActual_Diagnostics_String := 'F062 Sensor connection faulty';
   					16778254:
   						qActual_Diagnostics_String := 'F062 Sensor connection faulty';
   					16778256:
   						qActual_Diagnostics_String := 'F062 Sensor connection faulty';
   					16778279:
   						qActual_Diagnostics_String := 'F806 Loop diagnostics';
   					16778295:
   						qActual_Diagnostics_String := 'F272 Main electronics faulty';
   					16778476:
   						qActual_Diagnostics_String := 'F151 Sensor electronic failure';
   					16778478:
   						qActual_Diagnostics_String := 'F151 Sensor electronic failure';
   					16778479:
   						qActual_Diagnostics_String := 'F151 Sensor electronic failure';
   					16778480:
   						qActual_Diagnostics_String := 'F151 Sensor electronic failure';
   					16778490:
   						qActual_Diagnostics_String := 'F419 Power cycle required';
   					25165858:
   						qActual_Diagnostics_String := 'F062 Sensor connection faulty';
   					25165867:
   						qActual_Diagnostics_String := 'F801 Supply voltage too low';
   					25165875:
   						qActual_Diagnostics_String := 'F435 Linearization faulty';
   					25165891:
   						qActual_Diagnostics_String := 'F803 Loop current faulty';
   					25165918:
   						qActual_Diagnostics_String := 'F942 In safety distance';
   					25165920:
   						qActual_Diagnostics_String := 'F437 Configuration incompatible';
   					25165922:
   						qActual_Diagnostics_String := 'F282 Data storage inconsistent';
   					25165927:
   						qActual_Diagnostics_String := 'F242 Firmware incompatible';
   					25165931:
   						qActual_Diagnostics_String := 'F252 Module incompatible';
   					25165933:
   						qActual_Diagnostics_String := 'F270 Main electronics defective';
   					25165942:
   						qActual_Diagnostics_String := 'F941 Echo lost';
   					25165944:
   						qActual_Diagnostics_String := 'F270 Main electronics defective';
   					25165945:
   						qActual_Diagnostics_String := 'F272 Main electronics faulty';
   					25165948:
   						qActual_Diagnostics_String := 'F270 Main electronics defective';
   					25165949:
   						qActual_Diagnostics_String := 'F272 Main electronics faulty';
   					25165951:
   						qActual_Diagnostics_String := 'F270 Main electronics defective';
   					25165952:
   						qActual_Diagnostics_String := 'F270 Main electronics defective';
   					25165956:
   						qActual_Diagnostics_String := 'F270 Main electronics defective';
   					25165963:
   						qActual_Diagnostics_String := 'F410 Data transfer failed';
   					25165982:
   						qActual_Diagnostics_String := 'F283 Memory content inconsistent';
   					25165983:
   						qActual_Diagnostics_String := 'F270 Main electronics defective';
   					25165995:
   						qActual_Diagnostics_String := 'F270 Main electronics defective';
   					25165996:
   						qActual_Diagnostics_String := 'F151 Sensor electronic failure';
   					25165997:
   						qActual_Diagnostics_String := 'F805 Loop current faulty';
   					25165998:
   						qActual_Diagnostics_String := 'F151 Sensor electronic failure';
   					25166004:
   						qActual_Diagnostics_String := 'F151 Sensor electronic failure';
   					25166007:
   						qActual_Diagnostics_String := 'F151 Sensor electronic failure';
   					25166049:
   						qActual_Diagnostics_String := 'F283 Memory content inconsistent';
   					25166053:
   						qActual_Diagnostics_String := 'F273 Main electronics defective';
   					25166054:
   						qActual_Diagnostics_String := 'F388 Electronics and HistoROM defective';
   					25166424:
   						qActual_Diagnostics_String := 'F272 Main electronics faulty';
   					25166425:
   						qActual_Diagnostics_String := 'F151 Sensor electronic failure';
   					25166426:
   						qActual_Diagnostics_String := 'F151 Sensor electronic failure';
   					25166493:
   						qActual_Diagnostics_String := 'F151 Sensor electronic failure';
   					25166494:
   						qActual_Diagnostics_String := 'F151 Sensor electronic failure';
   					25166704:
   						qActual_Diagnostics_String := 'F168 Buildup detected';
   					25166705:
   						qActual_Diagnostics_String := 'F952 Foam detected';
   					25166799:
   						qActual_Diagnostics_String := 'F538 Configuration Sensor Unit invalid';
   					25166861:
   						qActual_Diagnostics_String := 'F062 Sensor connection faulty';
   					25166862:
   						qActual_Diagnostics_String := 'F062 Sensor connection faulty';
   					25166864:
   						qActual_Diagnostics_String := 'F062 Sensor connection faulty';
   					25166887:
   						qActual_Diagnostics_String := 'F806 Loop diagnostics';
   					25166903:
   						qActual_Diagnostics_String := 'F272 Main electronics faulty';
   					25167084:
   						qActual_Diagnostics_String := 'F151 Sensor electronic failure';
   					25167086:
   						qActual_Diagnostics_String := 'F151 Sensor electronic failure';
   					25167087:
   						qActual_Diagnostics_String := 'F151 Sensor electronic failure';
   					25167088:
   						qActual_Diagnostics_String := 'F151 Sensor electronic failure';
   					25167098:
   						qActual_Diagnostics_String := 'F419 Power cycle required';
   					33554446:
   						qActual_Diagnostics_String := 'C491 Current output simulation active';
   					33554526:
   						qActual_Diagnostics_String := 'C942 In safety distance';
   					33554547:
   						qActual_Diagnostics_String := 'C485 Process variable simulation active';
   					33554550:
   						qActual_Diagnostics_String := 'C941 Echo lost';
   					33554551:
   						qActual_Diagnostics_String := 'C485 Process variable simulation active';
   					33554575:
   						qActual_Diagnostics_String := 'C494 Switch output 1 simulation active';
   					33554576:
   						qActual_Diagnostics_String := 'C484 Failure mode simulation active';
   					33554656:
   						qActual_Diagnostics_String := 'C585 Simulation distance';
   					33554784:
   						qActual_Diagnostics_String := 'C586 Record map';
   					33554948:
   						qActual_Diagnostics_String := 'C412 Processing download';
   					33555312:
   						qActual_Diagnostics_String := 'C168 Buildup detected';
   					33555313:
   						qActual_Diagnostics_String := 'C952 Foam detected';
   					33555495:
   						qActual_Diagnostics_String := 'C806 Loop diagnostics';
   					33555889:
   						qActual_Diagnostics_String := 'C485 Process variable simulation active';
   					33555890:
   						qActual_Diagnostics_String := 'C485 Process variable simulation active';
   					33620111:
   						qActual_Diagnostics_String := 'C494 Switch output 2 simulation active';
   					41943054:
   						qActual_Diagnostics_String := 'C491 Current output simulation active';
   					41943134:
   						qActual_Diagnostics_String := 'C942 In safety distance';
   					41943155:
   						qActual_Diagnostics_String := 'C485 Process variable simulation active';
   					41943158:
   						qActual_Diagnostics_String := 'C941 Echo lost';
   					41943159:
   						qActual_Diagnostics_String := 'C485 Process variable simulation active';
   					41943183:
   						qActual_Diagnostics_String := 'C494 Switch output 1 simulation active';
   					41943184:
   						qActual_Diagnostics_String := 'C484 Failure mode simulation active';
   					41943264:
   						qActual_Diagnostics_String := 'C585 Simulation distance';
   					41943392:
   						qActual_Diagnostics_String := 'C586 Record map';
   					41943556:
   						qActual_Diagnostics_String := 'C412 Processing download';
   					41943920:
   						qActual_Diagnostics_String := 'C168 Buildup detected';
   					41943921:
   						qActual_Diagnostics_String := 'C952 Foam detected';
   					41944103:
   						qActual_Diagnostics_String := 'C806 Loop diagnostics';
   					41944497:
   						qActual_Diagnostics_String := 'C485 Process variable simulation active';
   					41944498:
   						qActual_Diagnostics_String := 'C485 Process variable simulation active';
   					42008719:
   						qActual_Diagnostics_String := 'C494 Switch output 2 simulation active';
   					67108868:
   						qActual_Diagnostics_String := 'M431 Trim required';
   					67108958:
   						qActual_Diagnostics_String := 'M942 In safety distance';
   					67108970:
   						qActual_Diagnostics_String := 'M438 Dataset different';
   					67108982:
   						qActual_Diagnostics_String := 'M941 Echo lost';
   					67109090:
   						qActual_Diagnostics_String := 'M287 Memory content inconsistent';
   					67109744:
   						qActual_Diagnostics_String := 'M168 Buildup detected';
   					67109745:
   						qActual_Diagnostics_String := 'M952 Foam detected';
   					67109896:
   						qActual_Diagnostics_String := 'M807 No Baseline due to insuf. volt. at 20 mA';
   					67109927:
   						qActual_Diagnostics_String := 'M806 Loop diagnostics';
   					67109944:
   						qActual_Diagnostics_String := 'M287 Memory content inconsistent';
   					75497476:
   						qActual_Diagnostics_String := 'M431 Trim required';
   					75497566:
   						qActual_Diagnostics_String := 'M942 In safety distance';
   					75497578:
   						qActual_Diagnostics_String := 'M438 Dataset different';
   					75497590:
   						qActual_Diagnostics_String := 'M941 Echo lost';
   					75497698:
   						qActual_Diagnostics_String := 'M287 Memory content inconsistent';
   					75498352:
   						qActual_Diagnostics_String := 'M168 Buildup detected';
   					75498353:
   						qActual_Diagnostics_String := 'M952 Foam detected';
   					75498504:
   						qActual_Diagnostics_String := 'M807 No Baseline due to insuf. volt. at 20 mA';
   					75498535:
   						qActual_Diagnostics_String := 'M806 Loop diagnostics';
   					75498552:
   						qActual_Diagnostics_String := 'M287 Memory content inconsistent';
   					134217772:
   						qActual_Diagnostics_String := 'S802 Supply voltage too high';
   					134217822:
   						qActual_Diagnostics_String := 'S942 In safety distance';
   					134217841:
   						qActual_Diagnostics_String := 'S968 Level limited';
   					134217846:
   						qActual_Diagnostics_String := 'S941 Echo lost';
   					134217863:
   						qActual_Diagnostics_String := 'S825 Electronics temperature';
   					134217881:
   						qActual_Diagnostics_String := 'S441 Current output saturated';
   					134218608:
   						qActual_Diagnostics_String := 'S168 Buildup detected';
   					134218609:
   						qActual_Diagnostics_String := 'S952 Foam detected';
   					134218639:
   						qActual_Diagnostics_String := 'S804 Switch output overloaded';
   					134218706:
   						qActual_Diagnostics_String := 'S826 Sensor temperature out of range';
   					134218791:
   						qActual_Diagnostics_String := 'S806 Loop diagnostics';
   					142606380:
   						qActual_Diagnostics_String := 'S802 Supply voltage too high';
   					142606430:
   						qActual_Diagnostics_String := 'S942 In safety distance';
   					142606449:
   						qActual_Diagnostics_String := 'S968 Level limited';
   					142606454:
   						qActual_Diagnostics_String := 'S941 Echo lost';
   					142606471:
   						qActual_Diagnostics_String := 'S825 Electronics temperature';
   					142606489:
   						qActual_Diagnostics_String := 'S441 Current output saturated';
   					142607216:
   						qActual_Diagnostics_String := 'S168 Buildup detected';
   					142607217:
   						qActual_Diagnostics_String := 'S952 Foam detected';
   					142607247:
   						qActual_Diagnostics_String := 'S804 Switch output overloaded';
   					142607314:
   						qActual_Diagnostics_String := 'S826 Sensor temperature out of range';
   					142607399:
   						qActual_Diagnostics_String := 'S806 Loop diagnostics';
   					536871006:
   						qActual_Diagnostics_String := '942 In safety distance';
   					536871030:
   						qActual_Diagnostics_String := '941 Echo lost';
   					536871262:
   						qActual_Diagnostics_String := '495 Diagnostic event simulation active';
   					536871792:
   						qActual_Diagnostics_String := '168 Buildup detected';
   					536871793:
   						qActual_Diagnostics_String := '952 Foam detected';
   					536871975:
   						qActual_Diagnostics_String := '806 Loop diagnostics';
   					545259614:
   						qActual_Diagnostics_String := '942 In safety distance';
   					545259638:
   						qActual_Diagnostics_String := '941 Echo lost';
   					545259870:
   						qActual_Diagnostics_String := '495 Diagnostic event simulation active';
   					545260400:
   						qActual_Diagnostics_String := '168 Buildup detected';
   					545260401:
   						qActual_Diagnostics_String := '952 Foam detected';
   					545260583:
   						qActual_Diagnostics_String := '806 Loop diagnostics';
   					16#9999:
   						qActual_Diagnostics_String := '';
   					else
   						qActual_Diagnostics_String := 'Error Code unknown';
   
   				end_case;
   
   				Trigger := FALSE;
   				DeviceData.OldState := DeviceData.State;
   		        DeviceData.State := DeviceData.State + 1;
   				DeviceData.CommSuccess := FALSE;
   				DeviceData.AcyclicData[0] := 0;
   				DeviceData.NewState := TRUE;
   
   
   
   			 elsif DeviceData.CommTimeOut then
   
   				temp_string1 := 'Error in step ';
   				Temp_DINT := DeviceData.State;
   				DTOS(Temp_DINT, temp_string2);
   				CONCAT(temp_string1, temp_string2, qAOI_Diagnostic_String);
   
   				DeviceData.OldState := DeviceData.State;
   				DeviceData.State := DeviceData.MaxState;
   				DeviceData.CommTimeOut := FALSE;
   				DeviceData.AcyclicData[0] := 0;
   				DeviceData.NewState := TRUE;
   
   		    end_if;
   
   		//*********************************
   	    91: // Last Diagnostic
   	    //*********************************
   
   		    CMD_Index := 298;
   			CMD_Subindex := 0;
   		    CMD_Wr := FALSE;
   			CMD_Rd := TRUE;
   			CMD_ByteLength := 4;
   			Trigger := TRUE;
   
   			if DeviceData.NewState then
   				DeviceData.StateDone := TRUE;
   			end_if;
   
   			if  DeviceData.CommSuccess and DeviceData.ReplayIndex = CMD_Index then
   
   				qLast_Diagnostics_Code	:= DeviceData.AcyclicData[0];
   
   				case qLast_Diagnostics_Code of
   
   					0:
   						qLast_Diagnostics_String := '--------';
   					16777250:
   						qLast_Diagnostics_String := 'F062 Sensor connection faulty';
   					16777259:
   						qLast_Diagnostics_String := 'F801 Supply voltage too low';
   					16777267:
   						qLast_Diagnostics_String := 'F435 Linearization faulty';
   					16777283:
   						qLast_Diagnostics_String := 'F803 Loop current faulty';
   					16777310:
   						qLast_Diagnostics_String := 'F942 In safety distance';
   					16777312:
   						qLast_Diagnostics_String := 'F437 Configuration incompatible';
   					16777314:
   						qLast_Diagnostics_String := 'F282 Data storage inconsistent';
   					16777319:
   						qLast_Diagnostics_String := 'F242 Firmware incompatible';
   					16777323:
   						qLast_Diagnostics_String := 'F252 Module incompatible';
   					16777325:
   						qLast_Diagnostics_String := 'F270 Main electronics defective';
   					16777334:
   						qLast_Diagnostics_String := 'F941 Echo lost';
   					16777336:
   						qLast_Diagnostics_String := 'F270 Main electronics defective';
   					16777337:
   						qLast_Diagnostics_String := 'F272 Main electronics faulty';
   					16777340:
   						qLast_Diagnostics_String := 'F270 Main electronics defective';
   					16777341:
   						qLast_Diagnostics_String := 'F272 Main electronics faulty';
   					16777343:
   						qLast_Diagnostics_String := 'F270 Main electronics defective';
   					16777344:
   						qLast_Diagnostics_String := 'F270 Main electronics defective';
   					16777348:
   						qLast_Diagnostics_String := 'F270 Main electronics defective';
   					16777355:
   						qLast_Diagnostics_String := 'F410 Data transfer failed';
   					16777374:
   						qLast_Diagnostics_String := 'F283 Memory content inconsistent';
   					16777375:
   						qLast_Diagnostics_String := 'F270 Main electronics defective';
   					16777387:
   						qLast_Diagnostics_String := 'F270 Main electronics defective';
   					16777388:
   						qLast_Diagnostics_String := 'F151 Sensor electronic failure';
   					16777389:
   						qLast_Diagnostics_String := 'F805 Loop current faulty';
   					16777390:
   						qLast_Diagnostics_String := 'F151 Sensor electronic failure';
   					16777396:
   						qLast_Diagnostics_String := 'F151 Sensor electronic failure';
   					16777399:
   						qLast_Diagnostics_String := 'F151 Sensor electronic failure';
   					16777441:
   						qLast_Diagnostics_String := 'F283 Memory content inconsistent';
   					16777445:
   						qLast_Diagnostics_String := 'F273 Main electronics defective';
   					16777446:
   						qLast_Diagnostics_String := 'F388 Electronics and HistoROM defective';
   					16777816:
   						qLast_Diagnostics_String := 'F272 Main electronics faulty';
   					16777817:
   						qLast_Diagnostics_String := 'F151 Sensor electronic failure';
   					16777818:
   						qLast_Diagnostics_String := 'F151 Sensor electronic failure';
   					16777885:
   						qLast_Diagnostics_String := 'F151 Sensor electronic failure';
   					16777886:
   						qLast_Diagnostics_String := 'F151 Sensor electronic failure';
   					16778096:
   						qLast_Diagnostics_String := 'F168 Buildup detected';
   					16778097:
   						qLast_Diagnostics_String := 'F952 Foam detected';
   					16778191:
   						qLast_Diagnostics_String := 'F538 Configuration Sensor Unit invalid';
   					16778253:
   						qLast_Diagnostics_String := 'F062 Sensor connection faulty';
   					16778254:
   						qLast_Diagnostics_String := 'F062 Sensor connection faulty';
   					16778256:
   						qLast_Diagnostics_String := 'F062 Sensor connection faulty';
   					16778279:
   						qLast_Diagnostics_String := 'F806 Loop diagnostics';
   					16778295:
   						qLast_Diagnostics_String := 'F272 Main electronics faulty';
   					16778476:
   						qLast_Diagnostics_String := 'F151 Sensor electronic failure';
   					16778478:
   						qLast_Diagnostics_String := 'F151 Sensor electronic failure';
   					16778479:
   						qLast_Diagnostics_String := 'F151 Sensor electronic failure';
   					16778480:
   						qLast_Diagnostics_String := 'F151 Sensor electronic failure';
   					16778490:
   						qLast_Diagnostics_String := 'F419 Power cycle required';
   					25165858:
   						qLast_Diagnostics_String := 'F062 Sensor connection faulty';
   					25165867:
   						qLast_Diagnostics_String := 'F801 Supply voltage too low';
   					25165875:
   						qLast_Diagnostics_String := 'F435 Linearization faulty';
   					25165891:
   						qLast_Diagnostics_String := 'F803 Loop current faulty';
   					25165918:
   						qLast_Diagnostics_String := 'F942 In safety distance';
   					25165920:
   						qLast_Diagnostics_String := 'F437 Configuration incompatible';
   					25165922:
   						qLast_Diagnostics_String := 'F282 Data storage inconsistent';
   					25165927:
   						qLast_Diagnostics_String := 'F242 Firmware incompatible';
   					25165931:
   						qLast_Diagnostics_String := 'F252 Module incompatible';
   					25165933:
   						qLast_Diagnostics_String := 'F270 Main electronics defective';
   					25165942:
   						qLast_Diagnostics_String := 'F941 Echo lost';
   					25165944:
   						qLast_Diagnostics_String := 'F270 Main electronics defective';
   					25165945:
   						qLast_Diagnostics_String := 'F272 Main electronics faulty';
   					25165948:
   						qLast_Diagnostics_String := 'F270 Main electronics defective';
   					25165949:
   						qLast_Diagnostics_String := 'F272 Main electronics faulty';
   					25165951:
   						qLast_Diagnostics_String := 'F270 Main electronics defective';
   					25165952:
   						qLast_Diagnostics_String := 'F270 Main electronics defective';
   					25165956:
   						qLast_Diagnostics_String := 'F270 Main electronics defective';
   					25165963:
   						qLast_Diagnostics_String := 'F410 Data transfer failed';
   					25165982:
   						qLast_Diagnostics_String := 'F283 Memory content inconsistent';
   					25165983:
   						qLast_Diagnostics_String := 'F270 Main electronics defective';
   					25165995:
   						qLast_Diagnostics_String := 'F270 Main electronics defective';
   					25165996:
   						qLast_Diagnostics_String := 'F151 Sensor electronic failure';
   					25165997:
   						qLast_Diagnostics_String := 'F805 Loop current faulty';
   					25165998:
   						qLast_Diagnostics_String := 'F151 Sensor electronic failure';
   					25166004:
   						qLast_Diagnostics_String := 'F151 Sensor electronic failure';
   					25166007:
   						qLast_Diagnostics_String := 'F151 Sensor electronic failure';
   					25166049:
   						qLast_Diagnostics_String := 'F283 Memory content inconsistent';
   					25166053:
   						qLast_Diagnostics_String := 'F273 Main electronics defective';
   					25166054:
   						qLast_Diagnostics_String := 'F388 Electronics and HistoROM defective';
   					25166424:
   						qLast_Diagnostics_String := 'F272 Main electronics faulty';
   					25166425:
   						qLast_Diagnostics_String := 'F151 Sensor electronic failure';
   					25166426:
   						qLast_Diagnostics_String := 'F151 Sensor electronic failure';
   					25166493:
   						qLast_Diagnostics_String := 'F151 Sensor electronic failure';
   					25166494:
   						qLast_Diagnostics_String := 'F151 Sensor electronic failure';
   					25166704:
   						qLast_Diagnostics_String := 'F168 Buildup detected';
   					25166705:
   						qLast_Diagnostics_String := 'F952 Foam detected';
   					25166799:
   						qLast_Diagnostics_String := 'F538 Configuration Sensor Unit invalid';
   					25166861:
   						qLast_Diagnostics_String := 'F062 Sensor connection faulty';
   					25166862:
   						qLast_Diagnostics_String := 'F062 Sensor connection faulty';
   					25166864:
   						qLast_Diagnostics_String := 'F062 Sensor connection faulty';
   					25166887:
   						qLast_Diagnostics_String := 'F806 Loop diagnostics';
   					25166903:
   						qLast_Diagnostics_String := 'F272 Main electronics faulty';
   					25167084:
   						qLast_Diagnostics_String := 'F151 Sensor electronic failure';
   					25167086:
   						qLast_Diagnostics_String := 'F151 Sensor electronic failure';
   					25167087:
   						qLast_Diagnostics_String := 'F151 Sensor electronic failure';
   					25167088:
   						qLast_Diagnostics_String := 'F151 Sensor electronic failure';
   					25167098:
   						qLast_Diagnostics_String := 'F419 Power cycle required';
   					33554446:
   						qLast_Diagnostics_String := 'C491 Current output simulation active';
   					33554526:
   						qLast_Diagnostics_String := 'C942 In safety distance';
   					33554547:
   						qLast_Diagnostics_String := 'C485 Process variable simulation active';
   					33554550:
   						qLast_Diagnostics_String := 'C941 Echo lost';
   					33554551:
   						qLast_Diagnostics_String := 'C485 Process variable simulation active';
   					33554575:
   						qLast_Diagnostics_String := 'C494 Switch output 1 simulation active';
   					33554576:
   						qLast_Diagnostics_String := 'C484 Failure mode simulation active';
   					33554656:
   						qLast_Diagnostics_String := 'C585 Simulation distance';
   					33554784:
   						qLast_Diagnostics_String := 'C586 Record map';
   					33554948:
   						qLast_Diagnostics_String := 'C412 Processing download';
   					33555312:
   						qLast_Diagnostics_String := 'C168 Buildup detected';
   					33555313:
   						qLast_Diagnostics_String := 'C952 Foam detected';
   					33555495:
   						qLast_Diagnostics_String := 'C806 Loop diagnostics';
   					33555889:
   						qLast_Diagnostics_String := 'C485 Process variable simulation active';
   					33555890:
   						qLast_Diagnostics_String := 'C485 Process variable simulation active';
   					33620111:
   						qLast_Diagnostics_String := 'C494 Switch output 2 simulation active';
   					41943054:
   						qLast_Diagnostics_String := 'C491 Current output simulation active';
   					41943134:
   						qLast_Diagnostics_String := 'C942 In safety distance';
   					41943155:
   						qLast_Diagnostics_String := 'C485 Process variable simulation active';
   					41943158:
   						qLast_Diagnostics_String := 'C941 Echo lost';
   					41943159:
   						qLast_Diagnostics_String := 'C485 Process variable simulation active';
   					41943183:
   						qLast_Diagnostics_String := 'C494 Switch output 1 simulation active';
   					41943184:
   						qLast_Diagnostics_String := 'C484 Failure mode simulation active';
   					41943264:
   						qLast_Diagnostics_String := 'C585 Simulation distance';
   					41943392:
   						qLast_Diagnostics_String := 'C586 Record map';
   					41943556:
   						qLast_Diagnostics_String := 'C412 Processing download';
   					41943920:
   						qLast_Diagnostics_String := 'C168 Buildup detected';
   					41943921:
   						qLast_Diagnostics_String := 'C952 Foam detected';
   					41944103:
   						qLast_Diagnostics_String := 'C806 Loop diagnostics';
   					41944497:
   						qLast_Diagnostics_String := 'C485 Process variable simulation active';
   					41944498:
   						qLast_Diagnostics_String := 'C485 Process variable simulation active';
   					42008719:
   						qLast_Diagnostics_String := 'C494 Switch output 2 simulation active';
   					67108868:
   						qLast_Diagnostics_String := 'M431 Trim required';
   					67108958:
   						qLast_Diagnostics_String := 'M942 In safety distance';
   					67108970:
   						qLast_Diagnostics_String := 'M438 Dataset different';
   					67108982:
   						qLast_Diagnostics_String := 'M941 Echo lost';
   					67109090:
   						qLast_Diagnostics_String := 'M287 Memory content inconsistent';
   					67109744:
   						qLast_Diagnostics_String := 'M168 Buildup detected';
   					67109745:
   						qLast_Diagnostics_String := 'M952 Foam detected';
   					67109896:
   						qLast_Diagnostics_String := 'M807 No Baseline due to insuf. volt. at 20 mA';
   					67109927:
   						qLast_Diagnostics_String := 'M806 Loop diagnostics';
   					67109944:
   						qLast_Diagnostics_String := 'M287 Memory content inconsistent';
   					75497476:
   						qLast_Diagnostics_String := 'M431 Trim required';
   					75497566:
   						qLast_Diagnostics_String := 'M942 In safety distance';
   					75497578:
   						qLast_Diagnostics_String := 'M438 Dataset different';
   					75497590:
   						qLast_Diagnostics_String := 'M941 Echo lost';
   					75497698:
   						qLast_Diagnostics_String := 'M287 Memory content inconsistent';
   					75498352:
   						qLast_Diagnostics_String := 'M168 Buildup detected';
   					75498353:
   						qLast_Diagnostics_String := 'M952 Foam detected';
   					75498504:
   						qLast_Diagnostics_String := 'M807 No Baseline due to insuf. volt. at 20 mA';
   					75498535:
   						qLast_Diagnostics_String := 'M806 Loop diagnostics';
   					75498552:
   						qLast_Diagnostics_String := 'M287 Memory content inconsistent';
   					134217772:
   						qLast_Diagnostics_String := 'S802 Supply voltage too high';
   					134217822:
   						qLast_Diagnostics_String := 'S942 In safety distance';
   					134217841:
   						qLast_Diagnostics_String := 'S968 Level limited';
   					134217846:
   						qLast_Diagnostics_String := 'S941 Echo lost';
   					134217863:
   						qLast_Diagnostics_String := 'S825 Electronics temperature';
   					134217881:
   						qLast_Diagnostics_String := 'S441 Current output saturated';
   					134218608:
   						qLast_Diagnostics_String := 'S168 Buildup detected';
   					134218609:
   						qLast_Diagnostics_String := 'S952 Foam detected';
   					134218639:
   						qLast_Diagnostics_String := 'S804 Switch output overloaded';
   					134218706:
   						qLast_Diagnostics_String := 'S826 Sensor temperature out of range';
   					134218791:
   						qLast_Diagnostics_String := 'S806 Loop diagnostics';
   					142606380:
   						qLast_Diagnostics_String := 'S802 Supply voltage too high';
   					142606430:
   						qLast_Diagnostics_String := 'S942 In safety distance';
   					142606449:
   						qLast_Diagnostics_String := 'S968 Level limited';
   					142606454:
   						qLast_Diagnostics_String := 'S941 Echo lost';
   					142606471:
   						qLast_Diagnostics_String := 'S825 Electronics temperature';
   					142606489:
   						qLast_Diagnostics_String := 'S441 Current output saturated';
   					142607216:
   						qLast_Diagnostics_String := 'S168 Buildup detected';
   					142607217:
   						qLast_Diagnostics_String := 'S952 Foam detected';
   					142607247:
   						qLast_Diagnostics_String := 'S804 Switch output overloaded';
   					142607314:
   						qLast_Diagnostics_String := 'S826 Sensor temperature out of range';
   					142607399:
   						qLast_Diagnostics_String := 'S806 Loop diagnostics';
   					536871006:
   						qLast_Diagnostics_String := '942 In safety distance';
   					536871030:
   						qLast_Diagnostics_String := '941 Echo lost';
   					536871262:
   						qLast_Diagnostics_String := '495 Diagnostic event simulation active';
   					536871792:
   						qLast_Diagnostics_String := '168 Buildup detected';
   					536871793:
   						qLast_Diagnostics_String := '952 Foam detected';
   					536871975:
   						qLast_Diagnostics_String := '806 Loop diagnostics';
   					545259614:
   						qLast_Diagnostics_String := '942 In safety distance';
   					545259638:
   						qLast_Diagnostics_String := '941 Echo lost';
   					545259870:
   						qLast_Diagnostics_String := '495 Diagnostic event simulation active';
   					545260400:
   						qLast_Diagnostics_String := '168 Buildup detected';
   					545260401:
   						qLast_Diagnostics_String := '952 Foam detected';
   					545260583:
   						qLast_Diagnostics_String := '806 Loop diagnostics';
   					else
   						qLast_Diagnostics_String := 'Error Code unknown';
   
   				end_case;
   
   				Trigger := FALSE;
   				DeviceData.OldState := DeviceData.State;
   		        DeviceData.State := DeviceData.State + 1;
   				DeviceData.CommSuccess := FALSE;
   				DeviceData.AcyclicData[0] := 0;
   				DeviceData.NewState := TRUE;
   
   			 elsif DeviceData.CommTimeOut then
   
   				temp_string1 := 'Error in step ';
   				Temp_DINT := DeviceData.State;
   				DTOS(Temp_DINT, temp_string2);
   				CONCAT(temp_string1, temp_string2, qAOI_Diagnostic_String);
   
   				DeviceData.OldState := DeviceData.State;
   		        DeviceData.State := DeviceData.MaxState;
   				DeviceData.CommTimeOut := FALSE;
   				DeviceData.AcyclicData[0] := 0;
   				DeviceData.NewState := TRUE;
   
   			end_if;
   
   		//*********************************
   		92: // Foam Index
   		//*********************************
   				CMD_Index := 8689;
   				CMD_Subindex := 0;
   				CMD_Wr := FALSE;
   				CMD_Rd := TRUE;
   				CMD_ByteLength := 4;
   				Trigger := TRUE;
   
   				if DeviceData.NewState then
   					DeviceData.StateDone := TRUE;
   				end_if;
   
   				if  DeviceData.CommSuccess and DeviceData.ReplayIndex = CMD_Index then
   
   					COP(DeviceData.AcyclicData[0], qFoamIndex, 1);
   
   					Trigger := FALSE;
   					DeviceData.OldState := DeviceData.State;
   					DeviceData.State := DeviceData.State + 1;
   					DeviceData.CommSuccess := FALSE;
   					DeviceData.AcyclicData[0] := 0;
   					DeviceData.NewState := TRUE;
   
   
   				 elsif DeviceData.CommTimeOut then
   
   					temp_string1 := 'Error in step ';
   					Temp_DINT := DeviceData.State;
   					DTOS(Temp_DINT, temp_string2);
   					CONCAT(temp_string1, temp_string2, qAOI_Diagnostic_String);
   
   					DeviceData.OldState := DeviceData.State;
   					DeviceData.State := DeviceData.MaxState;
   					DeviceData.CommTimeOut := FALSE;
   					DeviceData.AcyclicData[0] := 0;
   					DeviceData.NewState := TRUE;
   
   				end_if;
   
   		//*********************************
   		93: // Foam Detected
   		//*********************************
   				CMD_Index := 8716;
   				CMD_Subindex := 0;
   				CMD_Wr := FALSE;
   				CMD_Rd := TRUE;
   				CMD_ByteLength := 4;
   				Trigger := TRUE;
   
   				if DeviceData.NewState then
   
   					DeviceData.StateDone := TRUE;
   
   				end_if;
   
   				if  DeviceData.CommSuccess and DeviceData.ReplayIndex = CMD_Index then
   
   					COP(DeviceData.AcyclicData[0], qFoamDetectedREAL, 1);
   					qFoamDetected := qFoamDetectedREAL <> 0;
   
   					Trigger := FALSE;
   					DeviceData.OldState := DeviceData.State;
   					DeviceData.State := DeviceData.State + 1;
   					DeviceData.CommSuccess := FALSE;
   					DeviceData.AcyclicData[0] := 0;
   					DeviceData.NewState := TRUE;
   
   
   				 elsif DeviceData.CommTimeOut then
   
   					temp_string1 := 'Error in step ';
   					Temp_DINT := DeviceData.State;
   					DTOS(Temp_DINT, temp_string2);
   					CONCAT(temp_string1, temp_string2, qAOI_Diagnostic_String);
   
   					DeviceData.OldState := DeviceData.State;
   					DeviceData.State := DeviceData.MaxState;
   					DeviceData.CommTimeOut := FALSE;
   					DeviceData.AcyclicData[0] := 0;
   					DeviceData.NewState := TRUE;
   
   				end_if;
   
   		//*********************************
   		94: // Buildup Index
   		//*********************************
   				CMD_Index := 8700;
   				CMD_Subindex := 0;
   				CMD_Wr := FALSE;
   				CMD_Rd := TRUE;
   				CMD_ByteLength := 4;
   				Trigger := TRUE;
   
   				if DeviceData.NewState then
   					DeviceData.StateDone := TRUE;
   				end_if;
   
   				if  DeviceData.CommSuccess and DeviceData.ReplayIndex = CMD_Index then
   
   					COP(DeviceData.AcyclicData[0], qBuildupIndex, 1);
   
   					Trigger := FALSE;
   					DeviceData.OldState := DeviceData.State;
   					DeviceData.State := DeviceData.State + 1;
   					DeviceData.CommSuccess := FALSE;
   					DeviceData.AcyclicData[0] := 0;
   					DeviceData.NewState := TRUE;
   
   
   				 elsif DeviceData.CommTimeOut then
   
   					temp_string1 := 'Error in step ';
   					Temp_DINT := DeviceData.State;
   					DTOS(Temp_DINT, temp_string2);
   					CONCAT(temp_string1, temp_string2, qAOI_Diagnostic_String);
   
   					DeviceData.OldState := DeviceData.State;
   					DeviceData.State := DeviceData.MaxState;
   					DeviceData.CommTimeOut := FALSE;
   					DeviceData.AcyclicData[0] := 0;
   					DeviceData.NewState := TRUE;
   
   				end_if;
   
   		//*********************************
   		95: // Buildup Detected
   		//*********************************
   				CMD_Index := 8715;
   				CMD_Subindex := 0;
   				CMD_Wr := FALSE;
   				CMD_Rd := TRUE;
   				CMD_ByteLength := 4;
   				Trigger := TRUE;
   
   				if DeviceData.NewState then
   					DeviceData.StateDone := TRUE;
   				end_if;
   
   				if  DeviceData.CommSuccess and DeviceData.ReplayIndex = CMD_Index then
   
   					COP(DeviceData.AcyclicData[0], qBuildupDetectedREAL, 1);
   					qBuildupDetected := qBuildupDetectedREAL <> 0;
   
   					Trigger := FALSE;
   					DeviceData.OldState := DeviceData.State;
   					DeviceData.State := DeviceData.MaxState;
   					DeviceData.CommSuccess := FALSE;
   					DeviceData.AcyclicData[0] := 0;
   					DeviceData.NewState := TRUE;
   
   
   				 elsif DeviceData.CommTimeOut then
   
   					temp_string1 := 'Error in step ';
   					Temp_DINT := DeviceData.State;
   					DTOS(Temp_DINT, temp_string2);
   					CONCAT(temp_string1, temp_string2, qAOI_Diagnostic_String);
   
   					DeviceData.OldState := DeviceData.State;
   					DeviceData.State := DeviceData.MaxState;
   					DeviceData.CommTimeOut := FALSE;
   					DeviceData.AcyclicData[0] := 0;
   					DeviceData.NewState := TRUE;
   
   				end_if;
   
   		//*********************************
   		98: // End Step Trigger Guard
   		//*********************************
   
   				DeviceData.State := 0;
   				CommAOIBusy := 0;
   				DeviceAOISendRequest.[DeviceData.DevicePort] := 0;
   				ActiveComPort := 0;
   				ActiveAOI := 0;
   				DataToSend[0] := 0;
   				DataToSend[1] := 0;
   				DataToSend[2] := 0;
   				DataToSend[3] := 0;
   				DataToSend[4] := 0;
   				DataToSend[5] := 0;
    				DataToSend[6] := 0;
   				DataToSend[7] := 0;
    				DataToSend[8] := 0;
   				DataToSend[9] := 0;
   				DeviceData.StateDone := FALSE;
   				Skip := 0;
   				firstTimeDone := FALSE;
   				DeviceData.NewState := FALSE;
   				DeviceData.OldState := 0;
   				ActiveAOI := FALSE;
   
   				if SimActive then
   
   					SimActive := FALSE;
   					SimChanged := FALSE;
   
   				elsif UnitActive then
   
   					UnitActive := FALSE;
   					UnitChanged := FALSE;
   
   				elsif HeartbeatVerificationActive then
   
   					HeartbeatVerificationActive := FALSE;
   					HeartbeatVerificationChanged := FALSE;
   
   				elsif CondStatusActive then
   
   					CondStatusActive := FALSE;
   					CondStatusChanged := FALSE;
   
   				end_if;
   
   	end_case;
   
   	end_if;
   
   	//*************************
   	// Execution Area
   	//*************************
   	if DeviceData.State > StateMin and DeviceData.State < DeviceData.MaxState then
   
   		DataToSend[2] := DeviceData.DevicePort;
   		DataToSend[3] := CMD_Index;
   		DataToSend[4] := CMD_Subindex;
   		DataToSend[5].0 := CMD_Rd;
   		DataToSend[5].1 := CMD_Wr;
   		DataToSend[5].8 := CMD_ByteLength.0;  // Bits for the Length of the Data
   		DataToSend[5].9 := CMD_ByteLength.1;
   		DataToSend[5].10 := CMD_ByteLength.2;
   		DataToSend[5].11 := CMD_ByteLength.3;
   		DataToSend[5].12 := CMD_ByteLength.4;
   		DataToSend[5].13 := CMD_ByteLength.5;
   		DataToSend[5].14 := CMD_ByteLength.6;
   		DataToSend[5].15 := CMD_ByteLength.7;
   		DataToSend[5].7 := Trigger;
   
   		qCommError := CommError;
   
   	end_if;
   
   
   
   
   end_if;
END_ROUTINE
END_ADD_ON_INSTRUCTION
